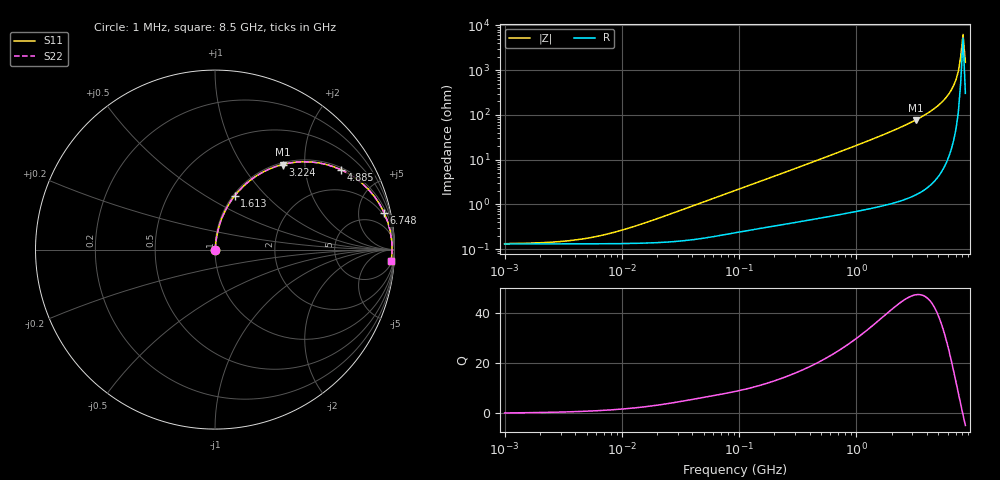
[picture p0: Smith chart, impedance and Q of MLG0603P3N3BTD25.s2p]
! S-Parameter Data Generated by TDK Corporation
! Copyright(C) 2025 TDK Corporation.
! All Rights Reserved.
! TDK P/N: MLG0603P3N3BTD25 (SMD / SMT Inductor (Coil))
! Property: L=3.3nH at 500MHz
! Size(LxWxT): 0.6x0.3x0.3mm
! Model Type: s2p (Touchstone File Format Version 1.0)
! Frequency: DC=Yes Start=1MHz Stop=8500MHz 198points Log-sweep
! Model Generated on Feb. 6, 2025
! Terms and conditions regarding TDK Simulation Models:
! 1)This simulation model is being provided solely for informational
!  purposes. Please refer to the specifications of the products in
!  terms of detailed characteristics of such products.
! 2)In no event shall TDK Corporation of any of its subsidiaries be
!  liable for any loss or damage arising, directly or indirectly,
!  from any information contained in this simulation model, including,
!  but not limited to loss or damages arising from any inaccuracies,
!  omissions or errors in connection with such information.
! 3)Any and all copyrights on this simulation model are owned by
!  TDK Corporation.  Duplication or redistribution of this simulation
!  model without prior written permission from TDK Corporation
!  is prohibited.
! 4)This simulation model is subject to any modification or change
!  without any prior notice.
! 5)Neither TDK Corporation nor any of its subsidiaries shall make any
!  warranty, express or implied, including but not limited to the
!  correctness, implied warranties of merchantability and fitness for
!  a particular purpose with respect to this simulation models.
! 6)The use of this simulation model shall be deemed to have consented
!  to the terms and conditions hereof.
! Port Assignments:
!  1 ---@@@--- 2
! Applicable Conditions:
!  Temperature = 25 degC
!  DC Bias Current = 0 A
!  Small Signal Operation
# Hz S MA R 50
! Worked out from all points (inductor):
!   197 points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, 1 MHz to 8.5 GHz, reference 50 ohm
!   read as one part in series: L = 3.62 nH near 18.32 MHz
!   highest Q = 47.4 at 3.224 GHz (marker M1), where L = 3.82 nH
!   self-resonance near 7.75 GHz
!   S11 on the Smith chart (normalised r, x): 1 MHz: 1.00, +0.00; 1.613 GHz: 1.02, +0.68; 3.224 GHz: 1.03, +1.55; 4.885 GHz: 1.08, +3.10; 6.748 GHz: 1.53, +9.03; 8.5 GHz: 7, -29
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1000000  0.001319 10.0  0.9987 -0.0  0.9987 -0.0  0.001319 10.0
2403882  0.001411 22.9  0.9987 -0.0  0.9987 -0.0  0.001411 22.9
4587603  0.001673 38.8  0.9987 -0.1  0.9987 -0.1  0.001673 38.8
9168677  0.002474 57.7  0.9987 -0.1  0.9987 -0.1  0.002474 57.7
2.10461e7  0.004987 73.5  0.9986 -0.3  0.9986 -0.3  0.004987 73.5
9.219544e7  0.02023 82.3  0.9975 -1.2  0.9975 -1.2  0.02023 82.3
4.229561e8  0.08733 82.0  0.9917 -5.0  0.9917 -5.0  0.08733 82.0
8.453103e8  0.1712 78.1  0.979 -9.9  0.979 -9.9  0.1712 78.1
1.613203e9  0.3199 69.8  0.939 -18.7  0.939 -18.7  0.3199 69.8
1.940355e9  0.3813 66.2  0.9152 -22.4  0.9152 -22.4  0.3813 66.2
2.559585e9  0.4934 59.2  0.859 -29.6  0.859 -29.6  0.4934 59.2
3.224109e9  0.6054 51.5  0.7832 -37.3  0.7832 -37.3  0.6054 51.5
4.061159e9  0.7304 41.8  0.6673 -46.9  0.6673 -46.9  0.7304 41.8
4.884749e9  0.831 32.4  0.5359 -56.2  0.5359 -56.2  0.831 32.4
5.87536e9  0.9184 21.4  0.3651 -66.6  0.3651 -66.6  0.9184 21.4
6.44363e9  0.9515 15.4  0.2658 -71.9  0.2658 -71.9  0.9515 15.4
6.748056e9  0.9645 12.3  0.2134 -74.3  0.2134 -74.3  0.9645 12.3
7.066863e9  0.9746 9.1  0.1594 -76.3  0.1594 -76.3  0.9746 9.1
7.400733e9  0.9818 6.0  0.1045 -77.0  0.1045 -77.0  0.9818 6.0
7.750377e9  0.9859 2.7  0.04947 -72.1  0.04947 -72.1  0.9859 2.7
8.116539e9  0.9868 -0.5  0.01575 32.6  0.01575 32.6  0.9868 -0.5
8.5e9  0.9844 -3.7  0.06624 74.5  0.06624 74.5  0.9844 -3.7
